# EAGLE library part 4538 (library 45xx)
Dual precision monostable MULTIVIBRATOR
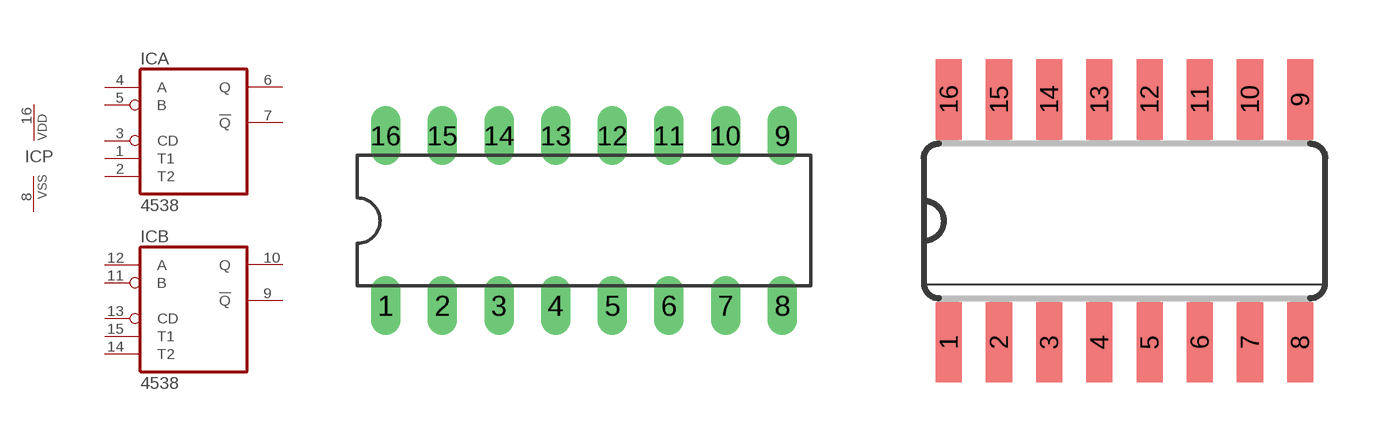
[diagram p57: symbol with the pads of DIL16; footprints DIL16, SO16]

Designator prefix IC; gates A=4528 B=4528 P=PWRN

## 4538N  [DIL16]
1  A:T1  in
2  A:T2  in
3  A:CD  in
4  A:A  in
5  A:B  in
6  A:Q  out
7  A:!Q  out
8  P:VSS  pwr
9  B:!Q  out
10  B:Q  out
11  B:B  in
12  B:A  in
13  B:CD  in
14  B:T2  in
15  B:T1  in
16  P:VDD  pwr

## 4538D  [SO16]
Pads as for DIL16

## Footprint DIL16 (pad centres in mm)
Dual In Line Package
drill 0.813 long: 1 -8.89,-3.81; 2 -6.35,-3.81; 3 -3.81,-3.81; 4 -1.27,-3.81; 5 1.27,-3.81; 6 3.81,-3.81; 7 6.35,-3.81; 8 8.89,-3.81; 9 8.89,3.81; 10 6.35,3.81; 11 3.81,3.81; 12 1.27,3.81; 13 -1.27,3.81; 14 -3.81,3.81; 15 -6.35,3.81; 16 -8.89,3.81

## Footprint SO16 (pad centres in mm)
Small Outline package 150 mil
smd 0.66 x 2.032: 1 -4.445,-3.073; 2 -3.175,-3.073; 3 -1.905,-3.073; 4 -0.635,-3.073; 5 0.635,-3.073; 6 1.905,-3.073; 7 3.175,-3.073; 8 4.445,-3.073; 9 4.445,3.073; 10 3.175,3.073; 11 1.905,3.073; 12 0.635,3.073; 13 -0.635,3.073; 14 -1.905,3.073; 15 -3.175,3.073; 16 -4.445,3.073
